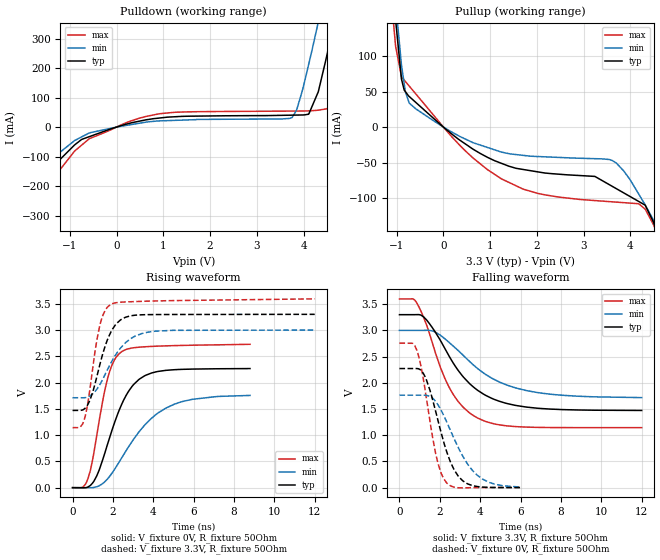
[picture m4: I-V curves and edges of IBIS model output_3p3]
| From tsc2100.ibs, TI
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|   output_3p3 Model
[Model]   output_3p3
Model_type   Output
Polarity   Non-Inverting
Vmeas = 1.65
Vref = 1.65
Cref = 10pF
Rref = 50
|   typ   min   max
|   (nom PVT)   (fast PVT)   (slow PVT)
|C_comp from frequency sweep method (F=13MHz)
|C_comp   3.792e-12   3.384e-12   4.175e-12
|ON state : BUFFER OUTPUT TURNED HIGH
|C_comp   3.792e-12   3.384e-12   4.175e-12
|OFF state: BUFFER OUTPUT TURNED LOW
|C_comp   2.682e-12   2.597e-12   2.696e-12
|C_comp from LC tank measurement(L=1nH)
|Resonant Frequency(Hz)   4.140e+09   4.170e+09   4.070e+09
C_comp   1.479e-12   1.458e-12   1.531e-12
|ON state : BUFFER OUTPUT TURNED HIGH
|Resonant Frequency(Hz)   4.140e+09   4.170e+09   4.070e+09
|C_comp   1.479e-12   1.458e-12   1.531e-12
|OFF state: BUFFER OUTPUT TURNED LOW
|Resonant Frequency(Hz)   4.380e+09   4.390e+09   4.370e+09
|C_comp   1.322e-12   1.316e-12   1.328e-12
| Where nom  PVT is Nominal Process, 3.3V, 26C
|   Fast PVT is Strong Process,  3.6V, -40C
|   Slow PVT is Weak Process,   3V, 86C
[Voltage Range]   3.3   3   3.6
|Ambient Temperature   25   85   -40
|Junction Temperature
[Temperature Range]   26   86   -40
[Pullup Reference]   3.3   3   3.6
[Pulldown Reference]   0   0   0
[Power Clamp Reference]   3.3   3   3.6
[GND Clamp Reference]   0   0   0
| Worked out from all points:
|   slope of the pulldown table from 0 to 0.495 V, typ, clamps not added: 24.5 ohm
|   slope of the pullup table from 0 to 0.495 V, typ, clamps not added: 19.8 ohm
|   falling waveform, V_fixture 3.3V, R_fixture 50Ohm: 20-80 % time 2.12ns typ, 2.67ns min, 1.59ns max; typ from 3.3 V to 1.47 V
|   rising waveform, V_fixture 0V, R_fixture 50Ohm: 20-80 % time 1.32ns typ, 2.09ns min, 815ps max; typ from 0 V to 2.27 V
|   rising waveform, V_fixture 3.3V, R_fixture 50Ohm: 20-80 % time 852ps typ, 1.22ns min, 597ps max; typ from 1.47 V to 3.3 V
|   falling waveform, V_fixture 0V, R_fixture 50Ohm: 20-80 % time 1.03ns typ, 1.41ns min, 734ps max; typ from 2.27 V to 0 V
[Pulldown]
|   Voltage   I(typ)   I(min)   I(max)
-3.3V     -1.746A    -1.562A    -1.945A
-2.131V   -589.6mA   -458.2mA   -738.7mA
-1.742V   -238.6mA   -175.6mA   -356.7mA
-1.505V   -156.6mA   -123mA     -204.3mA
-591mV    -32.99mA   -20.52mA   -40.6mA
939.6mV   31.03mA    21.05mA    45.54mA
3.753V    40.39mA    32.37mA    54.2mA
4.112V    43.64mA    213.6mA    54.93mA
4.314V    118.8mA    354.1mA    57.23mA
4.662V    365.9mA    608.7mA    123.1mA
5.072V    677.1mA    917.5mA    425.6mA
6.6V      1.891A     2.099A     1.69A
[Pullup]
|   Voltage   I(typ)   I(min)   I(max)
-3.3V     1.913A     1.903A     1.946A
-1.267V   313.1mA    346.3mA    292mA
-1.022V   150.6mA    175.2mA    113.9mA
-897.6mV  67.75mA    87.93mA    71.24mA
-732mV    43.14mA    33.78mA    57.89mA
633.6mV   -31.21mA   -22.03mA   -43.6mA
1.706V    -59.84mA   -39.94mA   -87.56mA
3.612V    -83.62mA   -47.14mA   -105.5mA
4.183V    -105.1mA   -95.07mA   -108.5mA
4.508V    -136.3mA   -133.1mA   -139.8mA
4.74V     -174.3mA   -175mA     -181.8mA
6.6V      -1.762A    -1.85A     -1.671A
[Ramp]
R_load = 50
|   typ   min   max
dV/dt_r   1.36213/1.3192e-09   1.05737/2.10733e-09   1.64818/8.23212e-10
dV/dt_f   1.09693/2.11336e-09   0.769883/2.66529e-09   1.47398/1.58809e-09
[Falling Waveform]
V_fixture = 3.3V
V_fixture_min = 3V
V_fixture_max = 3.6V
R_fixture = 50Ohm
|   Time   V(typ)   V(min)   V(max)
0s        3.3V       3V         3.6V
838ps     3.301V     3V         3.538V
1.394ns   3.176V     3.002V     3.049V
1.999ns   2.829V     2.915V     2.327V
2.457ns   2.512V     2.772V     1.919V
3.1ns     2.141V     2.546V     1.557V
3.864ns   1.859V     2.274V     1.329V
5.198ns   1.618V     1.975V     1.183V
6.807ns   1.515V     1.815V     1.149V
12ns      1.472V     1.717V     1.143V
[Rising Waveform]
V_fixture = 0V
V_fixture_min = 0V
V_fixture_max = 0V
R_fixture = 50Ohm
|   Time   V(typ)   V(min)   V(max)
0s        1.314nV    7.31nV     793.1pV
501ps     -2.578mV   -12.19uV   7.116mV
759ps     11.67mV    -2.27mV    167.6mV
1.195ns   221mV      16.66mV    981.2mV
1.746ns   842.1mV    171.5mV    2.091V
2.066ns   1.221V     340.1mV    2.424V
2.441ns   1.593V     571.4mV    2.591V
3.318ns   2.068V     1.074V     2.675V
4.635ns   2.234V     1.517V     2.7V
8.791ns   2.267V     1.756V     2.729V
[Rising Waveform]
V_fixture = 3.3V
V_fixture_min = 3V
V_fixture_max = 3.6V
R_fixture = 50Ohm
|   Time   V(typ)   V(min)   V(max)
0s        1.471V     1.712V     1.143V
382ps     1.47V      1.712V     1.156V
578ps     1.497V     1.712V     1.294V
873ps     1.679V     1.749V     1.91V
1.335ns   2.317V     1.952V     3.061V
1.604ns   2.681V     2.148V     3.366V
1.909ns   2.97V      2.38V      3.493V
2.623ns   3.244V     2.76V      3.535V
3.706ns   3.294V     2.958V     3.55V
12ns      3.3V       3V         3.594V
[Falling Waveform]
V_fixture = 0V
V_fixture_min = 0V
V_fixture_max = 0V
R_fixture = 50Ohm
|   Time   V(typ)   V(min)   V(max)
0s        2.272V     1.763V     2.757V
653ps     2.272V     1.763V     2.754V
862ps     2.272V     1.763V     2.622V
1.27ns    2.115V     1.763V     1.872V
1.781ns   1.475V     1.65V      675.9mV
2.074ns   1.037V     1.468V     269.2mV
2.348ns   677.1mV    1.248V     86.13mV
2.95ns    201.6mV    736.4mV    -4.87mV
3.849ns   19.35mV    238.1mV    -892.3uV
6.026ns   94.12uV    8.174mV    111.8uV
